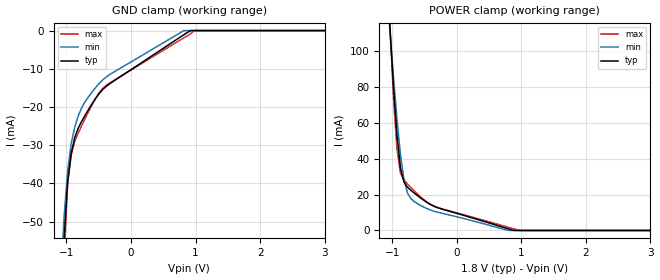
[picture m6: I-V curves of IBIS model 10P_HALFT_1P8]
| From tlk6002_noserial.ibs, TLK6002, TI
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[Model]   10P_HALFT_1P8
Model_type   Input
Polarity   Non-Inverting
Vinh =  1
Vinl =  0.8
C_comp   1.885425p   1.715283p   2.176444p
[Model Spec]
Vinh   1   0.91   1.09
Vinl   0.8   0.71   0.89
[Temperature Range]   25   125   -40
[Voltage Range]   1.8   1.62   1.98
[POWER_clamp]
-1.8V     655.3mA    532.6mA    788.8mA
-1.036V   113mA      111.2mA    114mA
-981.8mV  80.74mA    85.48mA    74.99mA
-927.3mV  53.3mA     62mA       45.23mA
-872.7mV  34.75mA    42.22mA    31.81mA
-818.2mV  26.87mA    28.19mA    28.08mA
-763.6mV  24.06mA    20.77mA    25.87mA
-600mV    19.15mA    14.71mA    19.94mA
-327.3mV  13.08mA    10.44mA    13.12mA
763.6mV   1.302mA    344.2uA    2.138mA
981.8mV   0A         0A         0A
3.6V      0A         0A         0A
[GND_clamp]
-1.8V     -583.5mA   -421.3mA   -777.4mA
-1.091V   -78.82mA   -65.78mA   -92.88mA
-1.036V   -54.59mA   -48.78mA   -59mA
-981.8mV  -39.57mA   -36.83mA   -40.23mA
-927.3mV  -32.19mA   -29.68mA   -32.69mA
-818.2mV  -25.56mA   -22.36mA   -26.86mA
-709.1mV  -22.12mA   -18.56mA   -22.97mA
-490.9mV  -16.43mA   -13.81mA   -16.21mA
-381.8mV  -14.58mA   -12.13mA   -14.31mA
818.2mV   -1.106mA   0A         -1.917mA
981.8mV   0A         0A         0A
3.6V      0A         0A         0A
